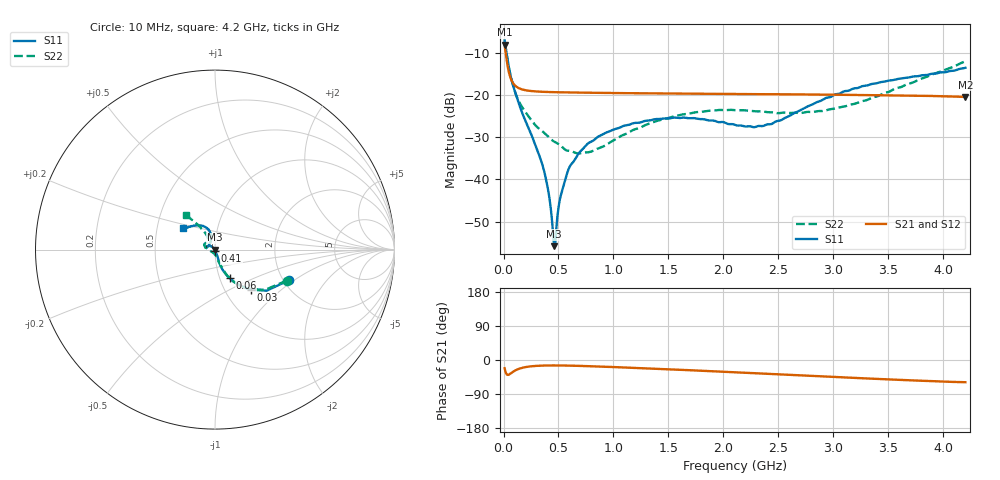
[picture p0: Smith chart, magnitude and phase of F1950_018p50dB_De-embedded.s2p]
! Integrated Device Technology
! Corporate Headquarters
! 6024 Silver Creek Valley Road
! San Jose, CA 95138  USA
! Phone:  1-408-284-8200
! Toll Free:  1-800-223-1366
! Webpage:  http://www.idt.com/
! Timing and RF Division
! 515 Groton Road, Suite 102
! Westford, MA 01886-6024
! Device:  F1950
! Description: 7-bit 0.25 dB Digital Step Attenuator
! Frequency:  150.0 -  4000.00 MHz
! Package:  4x4 mm Thin QFN Plastic Package: 24 pin
! Ports:  2 RF, 12 DC
!  Pin  1  = D0
!  Pin  2  = VDD
!  Pin  3  = Vmode
!  Pin  4  = GND
!  Pin  5  = RF1  =  Port 1
!  Pin  6  = GND
!  Pin  7  = GND
!  Pin  8  = GND
!  Pin  9  = GND
!  Pin 10  = GND
!  Pin 11  = GND
!  Pin 12  = GND
!  Pin 13  = GND
!  Pin 14  = RF2  =  Port 2
!  Pin 15  = GND
!  Pin 16  = LE
!  Pin 17  = CLK
!  Pin 18  = DATE
!  Pin 19  = D6
!  Pin 20  = D5
!  Pin 21  = D4
!  Pin 22  = D3
!  Pin 23  = D2
!  Pin 24  = D1
! State:  74
! Atten State:  18.50 dB
! Voltage:  +5.00 Volts
! Current:  Not Measured mA
! Data:  The device was measured on a the F195X evaluation board which has
!  individual transmission lines to the RF pins.  Data was collected
!  using a calibrated network analyzer.  The evaluation board was
!  de-embedded using a TRL calibration technique.
!  The reference plane is the edge of the package pin.
! Misc:  Board 2019
!  Action Tracker AT0250
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# GHz S dB R 50
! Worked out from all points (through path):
!   420 points, 10 MHz to 4.2 GHz, reference 50 ohm
!   highest |S21| = -8.03 dB at 10 MHz (marker M1); lowest = -20.4 dB at 4.2 GHz (marker M2)
!   group delay of S21, straight-line fit = 30.7 ps
!   lowest |S11| = -55.8 dB at 460 MHz (marker M3), VSWR 1.00, Z = 49.9 - j0.113 ohm
!   |S11| at or under -10 dB: 27.27 MHz to end of sweep
!   |S22| runs from -33.8 to -7.2 dB; largest |S21 - S12| = 0.00017
!   S11 on the Smith chart (normalised r, x): 10 MHz: 2.15, -0.91; 30 MHz: 1.32, -0.65; 60 MHz: 1.11, -0.37; 410 MHz: 1.00, -0.01; 4.2 GHz: 0.68, +0.17
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0.01  -6.99 -22.3  -8.03 -21.7  -8.02 -21.7  -7.21 -23.3
0.03  -10.49 -48.4  -11.85 -38.3  -11.85 -38.3  -10.65 -48.7
0.06  -14.92 -62.8  -15.58 -36.6  -15.59 -36.6  -14.82 -62.7
0.11  -19.61 -70.7  -17.82 -27.1  -17.82 -27.1  -19.59 -68.9
0.17  -24.19 -71.6  -18.62 -20.6  -18.62 -20.6  -22.86 -73.6
0.34  -35.40 -70.2  -19.16 -14.9  -19.16 -14.9  -28.27 -81.0
0.41  -43.12 -76.3  -19.23 -14.4  -19.24 -14.4  -29.93 -83.6
0.45  -52.67 -104.3  -19.27 -14.4  -19.27 -14.4  -30.85 -88.5
0.46  -55.84 -135.4  -19.27 -14.3  -19.27 -14.4  -31.01 -90.0
0.48  -51.72 158.3  -19.28 -14.4  -19.28 -14.4  -31.28 -92.5
0.52  -43.89 141.3  -19.30 -14.5  -19.30 -14.5  -31.94 -95.4
0.58  -38.39 135.7  -19.33 -14.8  -19.33 -14.8  -33.15 -105.4
0.71  -33.03 138.2  -19.38 -15.7  -19.38 -15.7  -33.70 -127.1
1  -28.16 148.3  -19.47 -18.6  -19.47 -18.6  -30.72 -168.6
1.41  -25.65 163.6  -19.57 -23.4  -19.57 -23.4  -25.98 169.8
1.73  -25.42 169.1  -19.63 -27.4  -19.63 -27.5  -24.10 161.0
2.11  -27.08 159.0  -19.70 -32.6  -19.70 -32.6  -23.55 152.0
2.43  -26.87 127.3  -19.76 -36.7  -19.76 -36.7  -24.03 142.9
2.81  -22.18 105.8  -19.82 -42.0  -19.82 -42.0  -24.00 128.8
3.1  -19.04 107.4  -19.89 -46.0  -19.88 -46.0  -22.68 122.6
3.51  -16.50 117.8  -20.00 -51.3  -20.00 -51.4  -19.13 120.9
4.2  -13.47 146.2  -20.41 -58.6  -20.40 -58.7  -11.95 129.9
